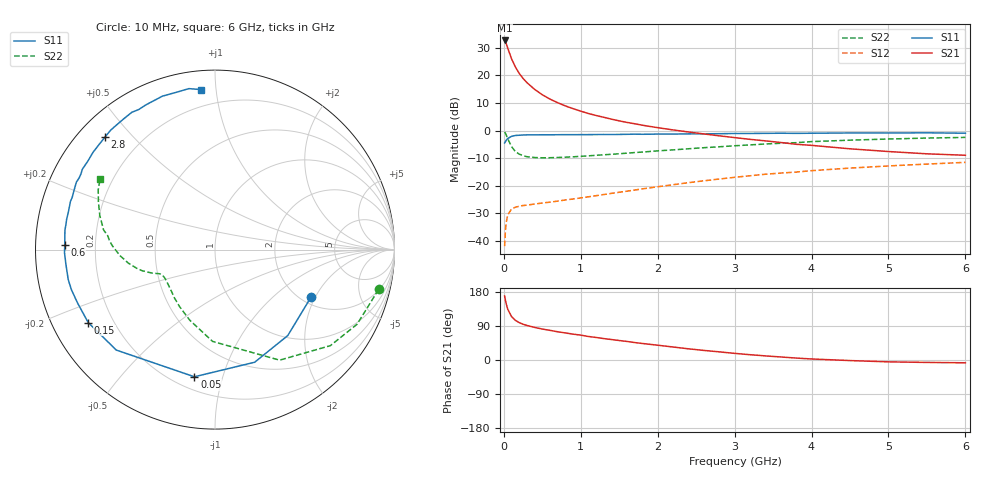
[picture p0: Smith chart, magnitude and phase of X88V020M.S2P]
! SIEMENS Small Signal Semiconductors
! BFP136W
! Si NPN RF Bipolar Junction Transistor in SOT343
! VCE = 8 V  IC = 20 mA
! Common Emitter S-Parameters:  September  1994
# GHz  S  MA  R  50
!  f  S11  S21  S12  S22
! GHz  MAG  ANG  MAG  ANG  MAG  ANG  MAG  ANG
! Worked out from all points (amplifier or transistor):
!   40 points, 10 MHz to 6 GHz, reference 50 ohm
!   highest |S21| = 32.6 dB at 10 MHz (marker M1)
!   |S21| within 3 dB of that: start of sweep to 53.72 MHz
!   unconditionally stable (mu >= 1): 957 MHz to 2.833 GHz
!   at 200 MHz: K = 0.31, MSG = 24.0 dB, |S12| = -27.4 dB
!   at 1.5 GHz: K = 1.15, MAG = 10.6 dB, |S12| = -22.3 dB
!   at 6 GHz: K = 0.96, MSG = 1.3 dB, |S12| = -11.5 dB
!   S11 on the Smith chart (normalised r, x): 10 MHz: 2.24, -1.85; 50 MHz: 0.28, -0.81; 150 MHz: 0.11, -0.26; 600 MHz: 0.09, +0.02; 2.8 GHz: 0.08, +0.42; 6 GHz: 0.10, +0.91
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0.01  0.5968 -26.5  42.57 168.8  0.0081 76.5  0.9381 -13.7
0.02  0.6276 -49.8  40.01 158.1  0.0148 70.2  0.8943 -27.7
0.03  0.6653 -70.6  37.59 149.1  0.0214 61.3  0.8362 -39.8
0.05  0.7178 -99.2  31.16 134.3  0.0295 48.3  0.7134 -59.7
0.1  0.7847 -134.5  19.89 114.5  0.0382 32.8  0.5118 -91.5
0.15  0.815 -150.1  14.1 104.7  0.0409 27.8  0.4176 -109.7
0.2  0.8213 -158.6  10.77 98.6  0.0428 25.2  0.3739 -121.9
0.25  0.8308 -164.5  8.746 94.4  0.044 24.6  0.3509 -130.2
0.3  0.8347 -168.5  7.349 91.2  0.0448 24.5  0.3364 -136.0
0.4  0.8348 -174.6  5.554 86.0  0.0468 26.0  0.3248 -143.9
0.5  0.8386 -178.8  4.438 81.7  0.0489 28.0  0.3213 -148.8
0.6  0.8376 178.1  3.699 78.2  0.0507 30.3  0.3223 -151.6
0.7  0.8397 175.0  3.186 74.5  0.0529 32.5  0.3253 -153.5
0.8  0.8432 172.6  2.786 71.4  0.0555 34.7  0.3297 -154.9
1.1  0.8435 165.4  2.031 62.0  0.0633 40.2  0.3485 -157.5
1.5  0.8501 158.1  1.495 51.4  0.0765 46.1  0.3807 -160.2
2.2  0.863 145.3  1.025 34.3  0.1047 49.6  0.4468 -166.4
2.8  0.8769 134.3  0.802 21.5  0.1327 48.7  0.5084 -173.8
3.2  0.8853 127.6  0.693 14.0  0.1519 46.4  0.5496 -179.2
4.5  0.9037 108.9  0.467 -1.5  0.2092 36.8  0.6695 163.5
5.5  0.9086 99.2  0.379 -6.4  0.2474 28.1  0.7309 152.9
6  0.8947 94.9  0.357 -7.4  0.2656 23.6  0.7511 148.5
